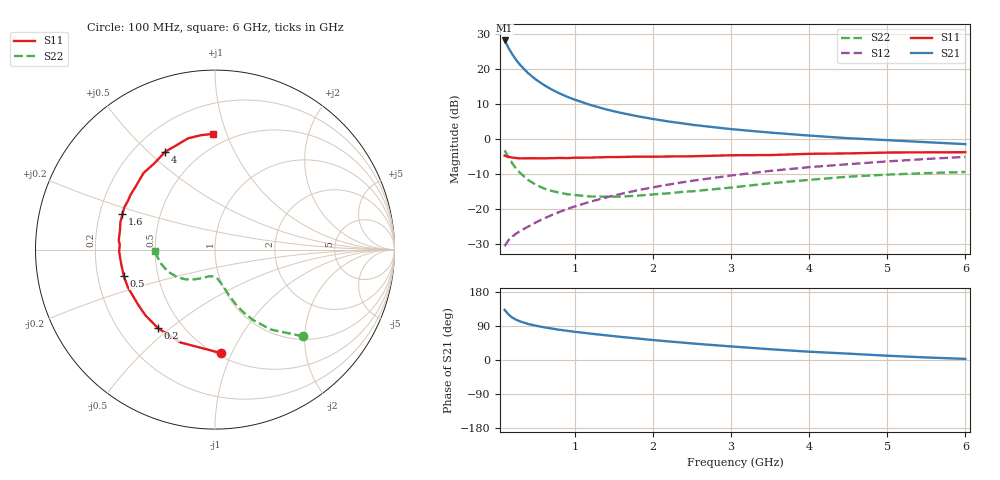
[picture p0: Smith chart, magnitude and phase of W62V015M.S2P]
! SIEMENS Small Signal Semiconductors
! BFR193W
! Si NPN RF Bipolar Junction Transistor in SOT323
! VCE = 2 V  IC = 15 mA
! Common Emitter S-Parameters:  September  1992
# GHz  S  MA  R  50
!  f  S11  S21  S12  S22
! GHz  MAG  ANG  MAG  ANG  MAG  ANG  MAG  ANG
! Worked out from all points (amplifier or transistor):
!   28 points, 100 MHz to 6 GHz, reference 50 ohm
!   highest |S21| = 28.1 dB at 100 MHz (marker M1)
!   |S21| within 3 dB of that: start of sweep to 173 MHz
!   unconditionally stable (mu >= 1): 819.9 MHz to 2.556 GHz
!   at 300 MHz: K = 0.69, MSG = 23.7 dB, |S12| = -26.3 dB
!   at 1.5 GHz: K = 1.04, MAG = 10.7 dB, |S12| = -16.2 dB
!   at 6 GHz: K = 0.91, MSG = 1.8 dB, |S12| = -5.1 dB
!   S11 on the Smith chart (normalised r, x): 100 MHz: 0.53, -0.91; 200 MHz: 0.37, -0.45; 500 MHz: 0.31, -0.13; 1.6 GHz: 0.30, +0.17; 4 GHz: 0.32, +0.57; 6 GHz: 0.41, +0.90
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0.1  0.5779 -86.5  25.31 132.3  0.0295 57.9  0.6882 -44.6
0.15  0.5521 -110.4  19.78 120.0  0.036 53.5  0.5429 -55.1
0.2  0.541 -125.9  15.96 111.7  0.0406 51.4  0.4445 -61.7
0.25  0.5331 -136.9  13.24 106.1  0.0447 52.1  0.3729 -66.3
0.3  0.5267 -144.7  11.3 101.7  0.0486 53.1  0.3256 -69.2
0.4  0.529 -156.6  8.668 95.2  0.056 55.6  0.2603 -73.4
0.5  0.5291 -164.0  7.025 90.5  0.0643 58.0  0.2215 -76.1
0.6  0.5281 -170.1  5.903 86.5  0.0731 60.1  0.1973 -79.1
0.7  0.5303 -174.7  5.07 83.0  0.0816 61.7  0.1815 -81.0
0.8  0.5343 -179.2  4.469 79.9  0.0906 62.9  0.1711 -83.4
0.9  0.5312 177.3  3.984 77.1  0.0998 63.8  0.1625 -85.0
1  0.5388 174.4  3.617 74.4  0.1089 64.4  0.1581 -87.0
1.2  0.5404 168.4  3.042 69.6  0.1273 65.0  0.1508 -91.8
1.4  0.5491 163.7  2.632 65.1  0.146 65.1  0.1498 -95.9
1.6  0.5522 159.1  2.335 60.8  0.1652 64.9  0.1504 -100.1
2.2  0.5608 147.0  1.77 49.0  0.2231 62.7  0.1674 -111.2
3  0.5836 133.0  1.377 35.8  0.3002 57.6  0.2021 -124.8
3.5  0.5877 125.1  1.229 28.4  0.3494 53.7  0.2328 -134.6
4  0.6119 116.9  1.114 21.9  0.3946 49.4  0.2603 -143.9
4.5  0.6202 110.0  1.022 16.8  0.4352 45.1  0.289 -154.7
5.5  0.6424 96.7  0.897 6.7  0.5164 36.3  0.3246 -173.1
6  0.6449 90.8  0.841 2.9  0.5535 31.7  0.3371 -179.0
